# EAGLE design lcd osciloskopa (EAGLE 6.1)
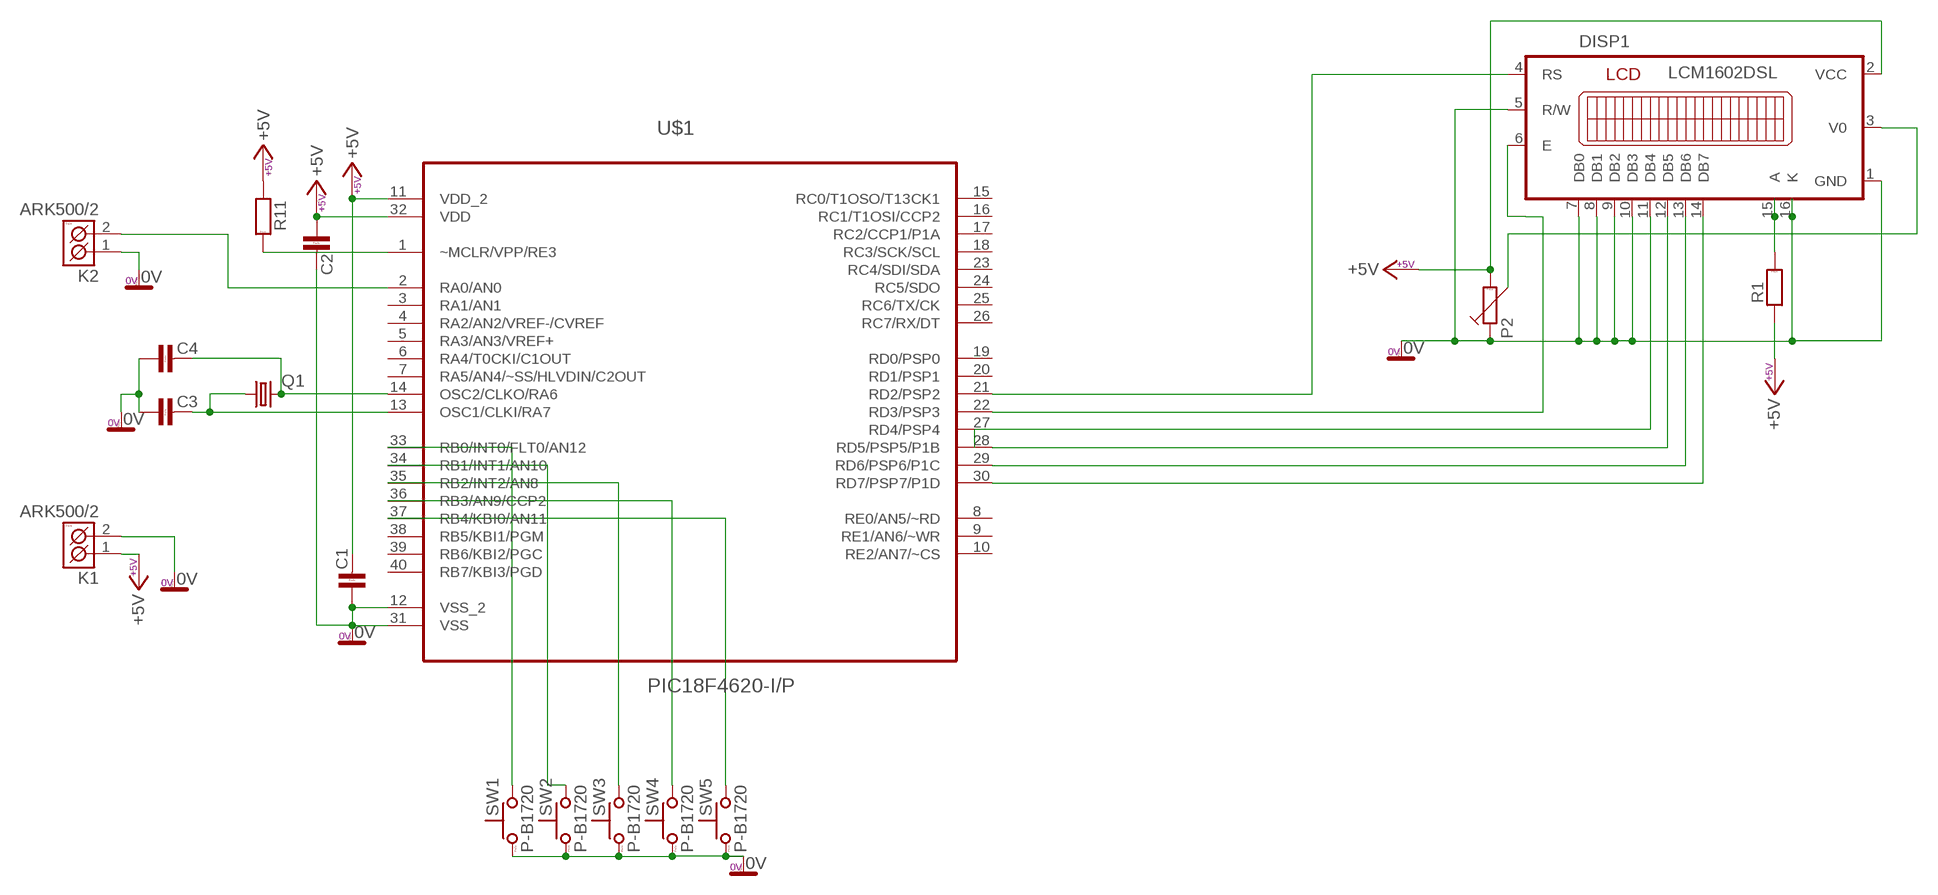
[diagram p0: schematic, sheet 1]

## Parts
C1  C-KERAMIK_7,5  [C-7,5]
C2  C-KERAMIK_7,5  [C-7,5]
C3  C-KERAMIK_7,5  [C-7,5]
C4  C-KERAMIK_7,5  [C-7,5]
DISP1  LCM1602DSL  [LCM1602DSL]
K1  ARK500/2  [ARK500/2]
K2  ARK500/2  [ARK500/2]
P2  TRIMRPT10V  [PT10V]
Q1  CRYSTALHC49U70  [HC49U70]
R1  R_7,5  [R-7,5]
R11  R_7,5  [R-7,5]
SW1  P-B1720  [P-B1720]
SW2  P-B1720  [P-B1720]
SW3  P-B1720  [P-B1720]
SW4  P-B1720  [P-B1720]
SW5  P-B1720  [P-B1720]
U$1  PIC18F4620-I/P  [DIP254P1524X635-40]

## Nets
+5V: C1.2 C2.1 DISP1.2(VCC) K1.1(K1) P2.2 R1.1 R11.1 U$1.11(VDD_2) U$1.32(VDD)
N$1: DISP1.4(RS) U$1.21(RD2/PSP2)
N$2: DISP1.6(E) U$1.22(RD3/PSP3)
N$3: DISP1.14(DB7) U$1.30(RD7/PSP7/P1D)
N$4: DISP1.13(DB6) U$1.29(RD6/PSP6/P1C)
N$5: DISP1.12(DB5) U$1.28(RD5/PSP5/P1B)
N$6: DISP1.11(DB4)
N$8: DISP1.3(V0) P2.3
N$9: SW5.2 U$1.37(RB4/KBI0/AN11)
N$10: SW4.2 U$1.36(RB3/AN9/CCP2)
N$11: SW3.2 U$1.35(RB2/INT2/AN8)
N$12: SW2.2 U$1.34(RB1/INT1/AN10)
N$13: SW1.2 U$1.33(RB0/INT0/FLT0/AN12)
N$17: K2.2(K2) U$1.2(RA0/AN0)
N$20: R11.2 U$1.1(~MCLR/VPP/RE3)
N$51: C3.2 Q1.1 U$1.13(OSC1/CLKI/RA7)
N$55: C4.2 Q1.2 U$1.14(OSC2/CLKO/RA6)
N$56: C1.1 C2.2 C3.1 C4.1 DISP1.1(GND) DISP1.5(R/W) DISP1.7(DB0) DISP1.8(DB1) DISP1.9(DB2) DISP1.10(DB3) DISP1.16(K) K1.2(K2) K2.1(K1) P2.1 SW1.1 SW2.1 SW3.1 SW4.1 SW5.1 U$1.12(VSS_2) U$1.31(VSS) ; supply symbol labelled 0V
N$57: DISP1.15(A) R1.2
Unconnected: SW1.3 SW1.4 SW2.3 SW2.4 SW3.3 SW3.4 SW4.3 SW4.4 SW5.3 SW5.4 U$1.3(RA1/AN1) U$1.4(RA2/AN2/VREF-/CVREF) U$1.5(RA3/AN3/VREF+) U$1.6(RA4/T0CKI/C1OUT) U$1.7(RA5/AN4/~SS/HLVDIN/C2OUT) U$1.8(RE0/AN5/~RD) U$1.9(RE1/AN6/~WR) U$1.10(RE2/AN7/~CS) U$1.15(RC0/T1OSO/T13CK1) U$1.16(RC1/T1OSI/CCP2) U$1.17(RC2/CCP1/P1A) U$1.18(RC3/SCK/SCL) U$1.19(RD0/PSP0) U$1.20(RD1/PSP1) U$1.23(RC4/SDI/SDA) U$1.24(RC5/SDO) U$1.25(RC6/TX/CK) U$1.26(RC7/RX/DT) U$1.27(RD4/PSP4) U$1.38(RB5/KBI1/PGM) U$1.39(RB6/KBI2/PGC) U$1.40(RB7/KBI3/PGD)

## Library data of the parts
C1-C4 = #PaJa_30:C-KERAMIK: Kondenzator - keramicky
DISP1 = #PaJa_displeje:LCM1602DSL: LCD - 2x16 + LED (TME - LCM1602DSL)
K1 K2 = #PaJa_konektory:ARK500/2: Svorkovnice - roztec 5mm - dvojita
P2 = #PaJa_30:TRIMR: Trimr
Q1 = crystal:CRYSTAL: CRYSTAL; OC_FARNELL: unknown; OC_NEWARK: unknown
R1 R11 = #PaJa_30:R: Rezistor
SW1-SW5 = #PaJa_prepinace:P-B1720: &micro;-tlacitko
U$1 = PIC18F4620:PIC18F4620-I/P: Flash Microcontrollers; MPN: PIC18F4620-I/P; OC_FARNELL: 1212704; OC_NEWARK: 89H0709; PACKAGE: DIP-40; SUPPLIER: Microchip

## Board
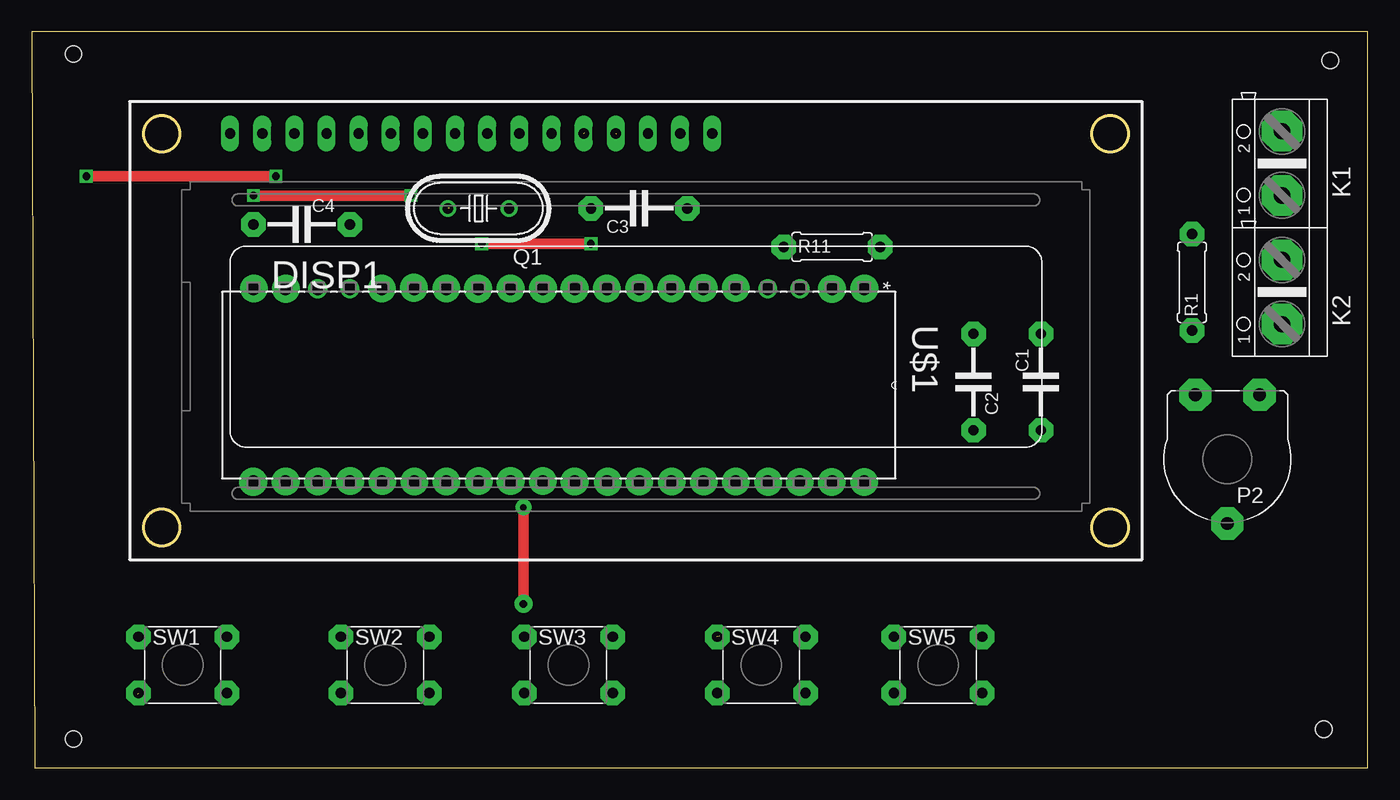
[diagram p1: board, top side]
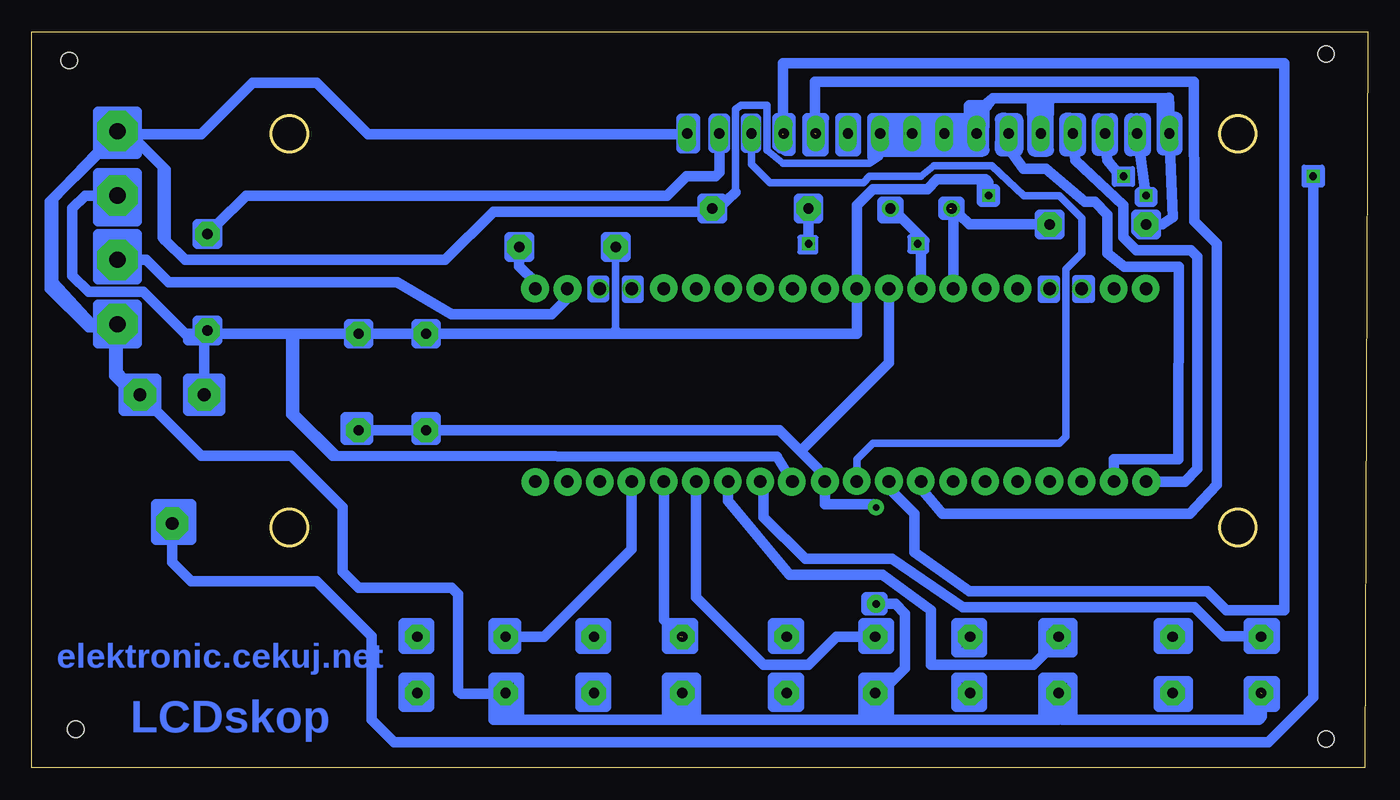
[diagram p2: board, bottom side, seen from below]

Size 105.59 x 58.16 mm. Coordinates in mm from the lower left corner, seen from the top.
Outline: 0.25,0 105.59,0 105.59,58.16 0,58.16 0.25,0
Copper layers (1*16): Top 0.035mm / dielectric 1.5mm / Bottom 0.035mm
Design rules: minimum track width 10mil, minimum drill 24mil, track to track 8mil, track to pad 8mil, pad to pad 8mil, via to via 8mil, smd to smd 8mil, copper to edge 40mil, drill to drill 8mil, minimum pad ring 10mil, minimum via ring 8mil, stop-mask expansion 4mil, vias tented up to drill 0mil, thermal gap 10mil
Holes 1.3 mm at 3.3,56.39 3.3,2.29 102.11,3.05 102.62,55.88

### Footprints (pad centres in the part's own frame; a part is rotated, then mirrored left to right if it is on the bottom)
C-7,5 = drill 0.813 pad 1.93 octagon: 1 -3.81,0; 2 3.81,0
LCM1602DSL = drill 0.813 pad 1.422 long: 1 -32.068,16.828; 2 -29.527,16.828; 3 -26.988,16.828; 4 -24.448,16.828; 5 -21.907,16.828; 6 -19.367,16.828; 7 -16.828,16.828; 8 -14.287,16.828; 9 -11.748,16.828; 10 -9.207,16.828; 11 -6.668,16.828; 12 -4.128,16.828; 13 -1.587,16.828; 14 0.953,16.828; 15 3.493,16.828; 16 6.032,16.828 | hole 2.8: -37.465,-14.287; 37.465,-14.287; 37.465,16.828; -37.465,16.828
ARK500/2 = drill 1.27 pad 3.2 octagon: 1 -2.54,0; 2 2.54,0
PT10V = drill 1.016 pad 2.54 octagon: 1 -2.54,-5.08; 2 2.54,-5.08; 3 0,5.08
HC49U70 = drill 0.813: 1 -2.413,0; 2 2.413,0
R-7,5 = drill 0.813 pad 1.93 octagon: 1 -3.81,0; 2 3.81,0
P-B1720 = drill 0.813 pad 1.93 octagon: 1 -3.493,-2.223; 2 -3.493,2.223; 3 3.493,-2.223; 4 3.493,2.223
DIP254P1524X635-40 = drill 0.991 square: 1 -15.24,48.26 | drill 0.991: 2 -15.24,45.72; 3 -15.24,43.18; 4 -15.24,40.64; 5 -15.24,38.1; 6 -15.24,35.56; 7 -15.24,33.02; 8 -15.24,30.48; 9 -15.24,27.94; 10 -15.24,25.4; 11 -15.24,22.86; 12 -15.24,20.32; 13 -15.24,17.78; 14 -15.24,15.24; 15 -15.24,12.7; 16 -15.24,10.16; 17 -15.24,7.62; 18 -15.24,5.08; 19 -15.24,2.54; 20 -15.24,0; 21 0,0; 22 0,2.54; 23 0,5.08; 24 0,7.62; 25 0,10.16; 26 0,12.7; 27 0,15.24; 28 0,17.78; 29 0,20.32; 30 0,22.86; 31 0,25.4; 32 0,27.94; 33 0,30.48; 34 0,33.02; 35 0,35.56; 36 0,38.1; 37 0,40.64; 38 0,43.18; 39 0,45.72; 40 0,48.26

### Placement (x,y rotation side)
C1  79.76,30.48 90 top
C2  74.42,30.48 270 top
C3  48.01,44.2 180 top
C4  21.34,42.93 0 top
DISP1  47.75,33.27 0 top
K1  98.81,47.75 90 top
K2  98.81,37.59 90 top
P2  94.49,24.38 180 top
Q1  35.31,44.2 180 top
R1  91.69,38.35 90 top
R11  63.25,41.15 0 top
SW1  11.94,8.13 0 top
SW2  27.94,8.13 0 top
SW3  42.42,8.13 0 top
SW4  57.66,8.13 0 top
SW5  71.63,8.13 0 top
U$1  17.53,22.61 270 top

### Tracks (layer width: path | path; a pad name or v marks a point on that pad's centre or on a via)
+5V  (via drill 0.5 pad 2.18, 0.6)
  Top 0.813: v17.53,45.21 v29.97,45.21
  Bottom 0.254: 92.46,34.04 R1.1 | 98.81,44.2 98.81,44.96 K1.1
  Bottom 0.61: R11.1 59.44,34.54 | C2.1 74.68,34.29
  Bottom 0.813: C1.2 74.68,34.29 74.42,34.54 C2.1 | 84.84,34.29 91.44,34.29 R1.1 | 92.46,34.04 92.96,34.04 | 93.22,34.04 96.77,37.59 101.09,37.59 102.36,38.86 102.36,44.2 101.35,45.21 99.06,45.21 98.81,44.96 | 91.95,30.73 91.95,34.29 R1.1 | 45.72,22.61 v45.52,22.61 U$1.32 46.71,24.59 81.53,24.64 | 59.44,34.54 59.69,34.29 C2.1 | 80.01,34.54 C1.2 | C1.2 84.84,34.29 | 84.84,34.29 85.09,34.04 85.09,27.94 81.79,24.64 81.53,24.64 | DISP1.2 v17.53,45.21 17.53,45.47 17.78,45.47 17.78,44.96 17.27,44.96 | U$1.11 40.39,44.45 39.12,45.72 34.8,45.72 34.04,46.48 30.23,46.48 29.97,46.23 29.97,45.72 | U$1.11 v40.41,37.85 40.64,37.85 | 81.53,24.64 84.84,27.94 84.84,34.29 | C1.2 C2.1 | C2.1 40.39,34.29 U$1.11 | P2.2 91.95,30.73 | 91.95,30.73 93.22,30.73 93.22,28.19 90.68,28.19 90.68,30.73 91.95,30.73 | R1.1 91.69,35.31 | 91.69,35.31 92.46,35.31 92.46,33.78 | 92.46,33.78 90.93,33.78 90.93,35.31 91.69,35.31 | 92.46,33.78 92.96,33.78 | 92.96,33.78 93.22,33.78 93.22,34.04 | 93.22,34.04 92.96,34.04 | 92.96,34.04 92.96,34.29 93.22,34.29 | 92.96,34.04 92.96,33.78 | C2.1 74.42,35.05 | 74.42,35.05 75.18,35.05 75.18,33.53 73.66,33.53 73.66,35.05 74.42,35.05 | C1.2 79.76,35.05 | 79.76,35.05 78.99,35.05 78.99,33.53 80.52,33.53 80.52,35.05 79.76,35.05 | R11.1 59.44,41.91 | 59.44,41.91 60.2,41.91 60.2,40.39 58.67,40.39 58.67,41.91 59.44,41.91 | v29.97,45.21 29.97,45.72 | 29.97,45.72 30.48,45.72 | 30.48,45.72 30.48,44.7 29.46,44.7 29.46,45.72 29.97,45.72 | 30.48,46.23 30.48,45.72 | 17.27,44.96 17.27,45.47 | 17.27,44.96 17.27,44.7 18.03,44.7 18.03,45.47 17.02,45.47 17.02,44.7
N$1  (via drill 0.5 pad 2.18)
  Bottom 0.813: 23.37,50.04 23.11,48.01 19.3,44.45 19.3,41.91 18.29,40.89 13.97,40.89 13.46,40.39 13.46,23.62 14.48,22.61 v17.5,22.61 U$1.21 | 23.37,50.04 23.11,50.04 | DISP1.4 23.37,50.04
N$2  (via drill 0.5 pad 2.18)
  Bottom 0.813: 28.19,49.28 28.26,50.1 DISP1.6 28.45,50.04 28.45,49.02 27.2,47.32 25.43,47.32 22.35,44.7 21.59,44.7 20.57,43.69 20.57,40.64 19.25,39.6 14.93,39.6 14.99,24.38 20.07,24.38 v20.07,22.63 U$1.22
N$3  (via drill 0.5 pad 2.18)
  Bottom 0.61: DISP1.14 48.7,47.69 47.24,46.23 39.88,46.23 39.37,46.74 35.31,46.74 34.29,47.57 29.72,47.57 27.18,45.21 24.38,45.21 22.61,43.43 22.61,40.64 23.88,39.37 23.88,26.16 24.38,25.65 39.12,25.65 40.39,24.38 v40.39,22.66 U$1.30
N$4  (1 unrouted)
  Bottom 0.813: U$1.29 37.85,22.1 35.81,20.07 35.81,17.02 31.5,13.97 12.7,13.97 11.18,12.45 6.6,12.45 6.6,55.68 46.23,55.68 46.23,50.04 46.48,49.78
N$5  (1 unrouted)
  Bottom 0.813: U$1.28 35.31,22.1 33.63,20.09 14.07,20.09 11.94,22.35 11.94,41.4 13.72,43.18 13.77,53.34 13.77,54.2 43.69,54.2 43.69,50.11 | 43.69,50.11 43.69,49.78 | 43.69,50.11 44.09,50.11 44.09,51.26
N$7
  Bottom 0.813: 44.2,44.45 44.2,44.96 | 44.2,44.96 44.96,44.96 44.96,43.43 43.43,43.43 43.43,44.96 44.2,44.96
N$8  (via drill 0.6)
  Top 0.813: v4.32,46.74 v19.3,46.74
  Bottom 0.813: v4.32,46.74 4.32,5.59 7.87,2.03 76.96,2.03 78.74,3.81 78.74,10.41 83.06,14.73 92.96,14.73 94.49,16.26 P2.3 94.49,20.57 | DISP1.3 20.83,50.04 20.57,48.01 19.56,46.74 v19.3,46.74 19.3,46.99 | 94.49,20.83 95.76,20.83 95.76,20.07 | 95.76,20.07 95.76,18.03 93.73,18.03 | 93.47,18.03 92.96,18.03 92.96,20.83 94.49,20.83 | 94.49,20.83 94.49,20.57 | 94.49,20.57 93.22,20.57 93.22,20.07 93.73,20.07 | 95.76,20.07 93.73,20.07 | 93.73,20.07 93.73,18.03 | 93.73,18.03 93.47,18.03 | 93.47,18.03 93.47,18.29 94.74,18.29 94.74,18.54 | 19.3,46.99 19.81,46.99 19.81,46.48 18.8,46.48 18.8,46.99 19.3,46.99
N$9
  Bottom 0.813: SW5.2 65.09,10.35 58.17,17.27 U$1.37
N$10  (1 unrouted)
  Bottom 0.813: U$1.36 55.63,11.68 54.36,10.41
N$11
  Bottom 0.813: U$1.35 53.09,14.48 53.09,14.22 53.09,13.46 47.75,8.13 44.2,8.13 41.97,10.35 SW3.2
N$12
  Bottom 0.813: U$1.34 50.55,21.08 45.72,15.24 38.35,15.24 34.54,12.45 34.54,8.13 26.42,8.13 24.38,10.16 24.45,10.22 SW2.2
N$13
  Bottom 0.813: U$1.33 47.75,22.86 47.75,19.81 44.45,16.51 37.59,16.51 32,12.7 13.72,12.7 11.43,10.41 8.64,10.41 | 8.64,10.41 8.64,11.43 | 8.64,11.43 9.4,11.43 9.4,9.4 7.62,9.4 | 7.62,9.4 7.62,11.43 | 7.62,11.43 8.13,11.43 8.64,11.43 | SW1.2 8.57,10.35 8.64,10.41 | 7.62,9.4 7.37,9.4 7.37,11.43 7.62,11.43
N$14
  Bottom 0.813: 25.15,43.18 25.15,43.69 | 25.15,43.69 25.91,43.69 25.91,42.16 24.38,42.16 24.38,43.69 25.15,43.69
N$15  (via drill 0.6 pad 1.42)
  other vias: 38.86,12.95
N$16
  Bottom 0.813: 51.21,49.02 50.8,49.02 | 50.8,49.02 50.8,49 | 50.8,49.02 50.8,51.28 51.66,51.28 51.66,51.21 51.69,51.21 51.69,49 51.11,49
N$17  (via drill 0.5 pad 2.18)
  Bottom 0.813: U$1.2 v63.25,37.82 63.25,37.08 64.52,35.81 72.39,35.81 76.71,38.35 94.74,38.35 96.52,40.13 K2.2 99.06,40.39
N$18  (via drill 0.5 pad 1.27)
  other vias: 38.86,20.57
N$20
  Bottom 0.813: U$1.1 65.79,38.35 67.06,39.62 67.06,40.64 67.06,40.89 | 67.06,40.89 67.31,41.15 R11.2 | 67.06,40.89 R11.2 | R11.2 67.06,41.91 | 67.06,41.91 66.29,41.91 66.29,40.39 67.82,40.39 67.82,41.91 67.06,41.91 | 67.06,40.89 R11.2
N$23
  Bottom 0.813: 8.89,10.92 8.89,11.18
N$24
  Bottom 0.813: 8.13,10.67 8.38,10.67 8.38,10.16 8.38,9.91
N$25
  Bottom 0.813: 8.13,10.41 8.64,10.41 8.64,10.16
N$26
  Bottom 0.813: 8.64,5.84 8.64,6.86 9.4,6.86 9.4,4.32 8.89,4.32 8.89,4.83
N$27
  Bottom 0.813: 8.64,4.83 7.37,4.83 7.37,6.86 8.38,6.86
N$28
  Bottom 0.813: 15.49,10.41 15.49,11.43 14.22,11.43 14.22,9.4 16.51,9.4 16.51,11.43 14.99,11.43 14.99,11.18
N$29
  Bottom 0.813: 14.99,10.16 15.49,10.16 15.49,9.91
N$30
  Bottom 0.813: 61.21,10.41 61.21,11.43 | 61.21,11.43 60.2,11.43 60.2,9.4 61.47,9.4 61.98,9.4 | 61.98,9.4 61.98,11.43 | 61.98,11.43 61.21,11.43 | 61.98,11.43 62.23,11.43 62.23,9.4 61.98,9.4
N$31
  Bottom 0.813: 14.48,6.1 14.73,6.1 14.73,5.33 15.49,5.33 | 15.49,5.33 16,5.33 16,6.1 14.99,6.1 14.99,6.35 15.49,6.35 15.49,6.1 15.49,5.33 | 15.49,4.83 14.22,4.83 14.22,6.86 16.51,6.86 16.51,4.83 15.49,4.83 | 15.49,4.83 15.49,5.33
N$32
  Bottom 0.813: 24.38,10.41 23.37,10.41 | 23.37,10.41 23.37,10.92 23.37,11.18 23.37,11.43 25.65,11.43 25.65,9.14 23.37,9.14 23.37,10.41
N$33
  Bottom 0.813: 24.64,6.1 24.64,7.11 | 25.15,7.11 25.65,7.11 25.65,5.08 | 25.65,5.08 24.64,5.08 | 24.64,5.08 23.37,5.08 23.37,7.11 24.64,7.11 | 24.64,7.11 25.15,7.11 | 25.15,7.11 25.15,6.1 24.89,6.1 24.89,5.33 | 25.65,5.08 25.65,4.32 23.37,4.32 23.37,4.83 24.64,4.83 24.64,5.08
N$34
  Bottom 0.813: 31.5,10.41 31.5,11.43 30.48,11.43 30.48,9.14 32.51,9.14 32.51,11.43 31.24,11.43 31.24,11.18
N$35
  Bottom 0.813: 31.24,10.41 31.5,10.41 31.5,9.91
N$36
  Bottom 0.813: 31.5,5.84 31.5,7.11 | 31.5,7.11 30.48,7.11 30.48,5.08 | 30.48,5.08 32.51,5.08 | 32.51,5.08 32.51,5.33 32.51,7.11 31.5,7.11 | 30.48,5.08 30.48,4.83 32.51,4.83 32.51,5.08
N$37
  Bottom 0.813: 39.12,10.41 38.86,10.41 38.86,11.43 37.85,11.43 37.85,9.4 39.88,9.4 39.88,11.43 39.12,11.43 39.12,11.18 39.12,10.92
N$38
  Bottom 0.813: 38.86,12.7 39.12,12.7 39.12,12.95
N$39
  Bottom 0.813: 45.97,5.84 45.97,7.11 | 45.97,7.11 44.96,7.11 44.96,4.83 46.23,4.83 46.74,4.83 | 46.74,4.83 46.74,7.11 | 46.74,7.11 45.97,7.11 | 46.74,7.11 46.99,7.11 46.99,4.83 46.74,4.83
N$40
  Bottom 0.813: 45.97,10.41 45.97,11.43 | 45.97,11.43 44.96,11.43 44.96,9.4 46.74,9.4 46.74,11.43 | 46.74,11.43 45.97,11.43 | 46.74,11.43 46.99,11.43 46.99,9.4
N$41
  Bottom 0.813: 54.1,6.1 54.1,7.11 | 54.1,7.11 53.59,7.11 53.34,7.11 | 53.34,7.11 53.34,4.32 | 53.34,4.32 55.12,4.32 55.12,7.11 | 55.12,7.11 54.1,7.11 | 55.12,7.11 55.37,7.11 55.37,4.32 | 53.34,4.32 53.09,4.32 53.09,7.11 53.34,7.11
N$42
  Bottom 0.813: 54.1,10.41 54.1,11.43 | 54.1,11.43 54.86,11.43 55.12,11.43 | 55.12,11.43 55.12,9.4 53.34,9.4 53.34,11.43 54.1,11.43 | 55.12,11.43 55.37,11.43 55.37,9.4
N$43
  Bottom 0.813: 61.21,6.1 61.21,7.11 62.23,7.11 62.23,4.83 60.2,4.83 60.2,7.11 61.47,7.11 61.47,5.59
N$44
  Bottom 0.813: 60.96,5.33 60.71,5.33 60.71,5.84 61.21,5.84 61.21,5.08
N$45
  Bottom 0.813: 68.07,10.41 68.07,11.43 | 68.07,11.43 67.31,11.43 67.31,9.4 69.09,9.4 69.09,11.43 68.07,11.43
N$46
  Bottom 0.813: 74.93,10.16 74.93,10.41 | 74.93,10.41 74.93,11.43 | 74.93,11.43 74.17,11.43 74.17,9.4 75.18,9.4 | 75.18,9.4 75.95,9.4 | 75.95,9.4 75.95,11.43 75.18,11.43 | 74.93,11.43 76.2,11.43 76.2,9.4 75.95,9.4 | 75.18,9.4 75.18,10.16 | 74.93,10.41 75.44,10.41 75.44,10.92 74.93,10.92 74.93,9.91
N$47
  Bottom 0.813: 75.18,5.84 75.18,7.11 | 75.18,7.11 74.93,7.11 74.17,7.11 74.17,4.83 76.2,4.83 76.2,7.11 75.18,7.11
N$48
  Bottom 0.813: 91.69,29.21 91.19,29.21 91.19,29.97 92.2,29.97 92.2,28.96 91.95,28.96
N$49
  Bottom 0.813: 90.93,28.7 92.71,28.7 92.71,30.23 92.96,30.23 92.96,29.72
N$50
  Bottom 0.813: 98.3,44.96 98.3,45.72
N$51  (via drill 0.6)
  Top 0.813: v44.2,41.4 v35.56,41.4
  Bottom 0.406: 44.25,41.45 44.2,41.45 44.2,41.91 | 44.2,41.91 44.83,41.91 | 44.83,41.91 44.88,41.91 44.88,40.77 43.61,40.77 43.61,41.86 44.83,41.86 44.83,41.91 | 44.2,41.91 43.61,41.91 43.61,41.88 44.02,41.88 44.02,41.4
  Bottom 0.813: 37.59,43.94 37.85,43.94 37.85,44.7 | 37.85,44.7 37.08,44.7 37.08,43.69 | U$1.13 35.31,41.91 | C3.2 44.2,41.91 v44.2,41.4 | v35.56,41.4 35.05,41.66 35.31,41.91 | 35.31,41.91 37.08,43.69 | 37.08,43.69 37.59,44.2 Q1.1 | 37.08,43.69 37.08,43.43 38.35,43.43 38.35,44.7 37.85,44.7
N$52
  Bottom 0.813: 98.81,39.88 98.81,41.66 100.33,41.66 | 100.33,41.66 100.33,38.61 97.28,38.61 97.28,41.66 | 97.28,41.66 98.55,41.66 | 97.28,41.66 97.28,42.16 100.33,42.16 100.33,41.66
N$53
  Bottom 0.813: 99.31,40.13 99.06,40.13 99.06,39.37 98.55,39.37 | 98.55,39.37 98.3,39.37 98.3,39.62 98.55,39.62 98.55,39.37
N$54
  Bottom 0.813: 98.81,45.47 98.81,46.74 100.08,46.74 100.08,43.69 | 100.08,43.69 97.54,43.69 | 97.54,43.69 97.54,46.74 99.06,46.74 99.06,46.48 | 97.54,43.69 97.54,43.43 | 97.54,43.18 100.08,43.18 100.08,43.69 | 98.04,43.43 97.54,43.43 | 97.54,43.43 97.54,43.18 | 97.54,43.18 97.28,43.18 97.28,46.74 | 97.28,46.74 100.33,46.74 | 100.33,46.74 100.33,43.18 | 97.28,46.74 97.28,46.99 100.33,46.99 100.33,46.74
N$55  (via drill 0.5 pad 2.18)  (1 unrouted)
  Bottom 0.813: 33.02,44.2 33.02,44.7 32.26,44.7 32.26,43.69 | C4.2 31.5,42.93 32.26,43.69 | 32.26,43.69 32.77,44.2 v32.77,37.87 U$1.14 | 32.26,43.69 33.27,43.69 33.27,44.7 33.53,44.7 33.53,43.69
N$56  (via drill 0.5 pad 1.27)  (1 unrouted)
  Top 0.813: v38.86,20.57 v38.86,12.95
  Bottom 0.254: 54.36,6.1 SW4.1 | 68.33,6.1 SW5.1 | 53.85,50.04 DISP1.16 | 98.81,49.28 98.81,49.78 98.81,50.04 K1.2 | 100.08,34.04 98.81,34.04 98.81,34.29 K2.1
  Bottom 0.61: 49.99,45.47 49.96,52.05 49.53,52.32 47.5,52.32 47.5,48.77 46.23,47.75 39.37,47.75 38.61,48.26 38.61,50.04 DISP1.10
  Bottom 0.813: 98.55,50.8 99.57,50.8 99.57,50.29 98.3,50.29 98.3,49.78 98.04,49.78 98.04,48.77 | 98.81,50.55 98.81,51.82 | 98.81,51.82 100.33,51.82 100.33,48.77 98.55,48.77 | 98.04,48.77 97.54,48.77 97.54,51.56 | 97.54,51.56 97.54,51.82 98.81,51.82 | 97.54,51.56 97.28,51.56 | 97.28,51.56 97.28,51.82 | 97.28,51.56 97.28,48.51 98.55,48.51 | 100.08,34.8 100.08,36.32 | 100.08,36.58 97.28,36.58 97.28,33.53 100.08,33.53 100.08,34.8 | 96.52,29.97 97.54,29.97 97.54,28.45 96.77,28.45 96.77,28.7 96.01,28.7 96.01,29.72 96.77,29.72 96.77,29.21 | 68.07,3.81 68.07,5.91 SW5.1 68.2,5.84 68.33,5.84 | 68.07,3.81 54.36,3.81 | 54.36,3.81 54.17,3.81 | 54.17,3.81 SW4.1 54.36,5.91 54.36,3.81 | 54.17,3.81 38.93,3.81 SW3.1 38.86,5.91 | 38.86,5.91 38.86,5.84 | 38.86,5.84 38.86,3.81 24.45,3.81 SW2.1 24.45,4.13 24.13,3.81 8.64,3.81 8.38,4.06 8.38,5.84 | v38.86,20.57 39.12,20.83 42.9,20.83 42.9,22.89 42.93,22.89 U$1.31 42.75,22.66 43.51,23.67 43.69,23.88 44.83,25.02 | 38.86,5.84 38.61,6.1 38.35,6.1 36.58,7.87 36.58,12.19 37.34,12.95 v38.86,12.95 38.86,13.46 39.62,13.46 39.62,12.45 38.35,12.45 38.35,13.46 38.61,13.46 | 25.6,52.91 25.91,50.16 | 25.91,50.16 DISP1.5 26.1,52.13 25.6,52.91 | 38.61,50.04 38.35,50.04 38.42,50.1 DISP1.10 DISP1.9 DISP1.8 DISP1.7 30.91,50.1 30.91,50.67 | 98.3,50.04 98.81,49.78 | 98.81,34.04 98.81,31.24 98.3,30.73 | 98.3,30.73 P2.1 97.03,29.97 | C2.2 79.5,26.67 79.76,26.42 80.01,26.67 C1.1 | C1.1 C2.2 | C2.2 46.48,26.67 44.83,25.02 | 25.6,52.91 15.72,52.93 15.68,52.26 DISP1.1 15.43,43.5 16.26,42.93 C4.1 17.53,43.69 | K2.1 100.84,35.05 103.89,38.35 103.89,44.96 K1.2 | 98.3,50.04 98.81,50.04 99.31,50.04 99.31,49.53 100.33,48.51
  Bottom 0.813: 98.3,50.04 97.79,50.04 | 95.25,47.5 95.25,41.91 95,41.66 | C3.1 52.07,43.94 69.09,43.94 72.9,40.13 93.47,40.13 95,41.66 | C3.1 51.31,44.2 49.99,45.47 | 95,41.66 95,47.24 95.25,47.5 | 95.25,47.5 97.79,50.04 | 100.33,48.51 104.14,44.7 104.14,37.85 101.09,34.8 100.33,34.8 | 100.08,34.8 99.06,34.8 | 99.06,34.8 99.06,34.54 | 99.06,34.54 99.06,30.99 97.28,29.21 96.77,29.21 | 96.77,29.21 95.76,28.19 | 95.76,28.19 92.2,24.64 85.09,24.64 81.03,20.57 81.03,15.49 79.76,14.22 72.39,14.22 71.88,13.72 71.88,6.1 71.63,5.84 68.33,5.84 | U$1.12 37.85,32 44.83,25.02 | 53.85,50.04 78.99,50.04 83.06,54.1 88.14,54.1 92.2,50.04 97.79,50.04 | 38.86,5.91 38.86,7.11 | 38.86,7.11 38.61,7.11 | 38.61,7.11 38.1,7.11 | 38.1,7.11 37.59,7.11 | 38.1,7.11 38.1,4.32 37.85,4.32 37.85,6.35 38.61,6.35 38.61,7.11 | 38.86,7.11 39.88,7.11 39.88,4.32 39.12,4.32 39.12,4.83 39.37,4.83 39.37,6.35 | 68.33,5.84 68.33,7.11 | 68.33,7.11 67.06,7.11 67.06,5.08 | 67.06,4.83 67.06,4.32 69.09,4.32 | 69.09,4.32 69.09,7.11 68.33,7.11 | 68.33,5.84 68.33,4.83 67.06,4.83 | 67.06,4.83 67.06,5.08 | 67.06,5.08 67.31,5.08 | 68.07,3.81 69.09,3.81 69.09,4.32 | C1.1 79.76,27.69 80.77,27.69 80.77,25.91 78.99,25.91 78.99,27.69 79.5,27.69 | C2.2 74.42,27.69 75.18,27.69 75.18,25.91 73.66,25.91 73.66,27.69 74.17,27.69 | 97.03,29.97 97.03,30.73 | 97.03,30.73 95.76,30.73 95.76,28.19 | 95.76,28.19 98.3,28.19 98.3,30.73 | 98.3,30.73 97.03,30.73 | 96.77,29.21 96.27,29.21 96.27,29.97 97.03,29.97 | 100.08,34.8 100.33,34.8 | 100.33,34.8 100.33,36.58 100.08,36.58 | 100.08,36.58 100.08,36.32 | 100.08,36.32 100.33,36.32 100.33,33.53 98.3,33.53 98.3,35.56 99.06,35.56 99.06,34.8
  Bottom 0.813: 99.06,34.54 98.81,34.54 98.81,34.29 | 100.33,48.51 98.55,48.51 | 98.55,48.51 98.55,49.53 | 98.04,48.77 98.55,48.77 | 98.55,48.77 98.55,50.55 | C3.1 51.82,44.96 | 51.82,44.96 52.58,44.96 52.58,43.43 51.05,43.43 51.05,44.96 51.82,44.96 | 17.53,43.69 18.29,43.69 18.29,42.42 18.03,42.16 16.76,42.16 16.76,43.69 17.53,43.69 | 25.91,50.16 25.73,50.16 25.73,52.3 25.86,52.3 25.45,52.91 29.62,52.91 | 29.62,52.91 30.3,52.32 | 30.3,52.32 30.3,50.67 30.91,50.67 | 30.91,50.67 31.04,50.67 31.04,50.09 | 30.1,52.25 30.1,52.3 29.62,52.91 | 30.3,52.32 31.5,52.32 31.52,52.3 31.52,50.34 31.62,50.24 31.62,51.28 30.94,51.97 30.94,50.98 31.04,50.88 31.04,51.44 31.01,51.44 30.81,51.23 30.81,51.28 30.79,51.31 | 30.46,51.21 30.56,51.21 30.56,51.11 30.58,51.11 30.58,51.41 | 30.46,51.74 30.4,51.74 30.4,51.69 30.38,51.69 30.38,51.41 30.58,51.41 | 30.58,51.41 30.61,51.41 30.73,51.41 30.73,51.03 30.76,51.03 30.76,50.62 | 30.61,51.31 30.79,51.31 | 30.79,51.31 30.94,51.31 30.94,50.44 30.96,50.44 30.96,50.11 30.91,50.11 30.91,50.14 30.81,50.14 30.81,50.49 | 30.79,51.31 30.79,51.33 39.14,51.33 39.14,49.78 | 39.14,48.26 39.14,49.78 | 39.14,49.78 37.92,51 37.92,50.65 37.8,50.52 32.49,50.52 32.26,50.75 32.26,50.6 31.04,49.38 37.64,49.38 37.85,49.58
  Bottom 1.016: 30.96,51.13 30.94,51.16 30.4,51.16 | 38.96,51.16 38.99,51.13 38.99,48.82 38.96,48.79 30.4,48.79 30.4,51.16 | 30.58,51.44 30.61,51.41 30.61,51.31 30.61,51.28 30.46,51.13 30.46,51.21 30.4,51.16
N$57
  Bottom 0.813: 91.69,42.42 91.69,42.93 | 91.69,42.93 92.46,42.93 92.46,41.4 90.93,41.4 90.93,42.93 | DISP1.15 51.25,47.05 51.56,46.74 53.85,46.74 55.37,45.21 88.65,45.21 90.93,42.93 | 90.93,42.93 R1.2 | 90.93,42.93 91.19,42.93 91.44,42.93 91.69,42.93
N$58
  Bottom 0.813: 53.77,50.09 53.77,51.26 53.19,51.26 53.19,48.95 54.23,48.95 54.23,51.21 53.85,51.21 | 53.8,51.21 53.85,51.21 | 53.85,51.21 53.85,51.26 | 53.85,51.26 54.23,51.26 | 53.85,51.26 53.75,51.26 53.75,51.16 | 53.75,51.13 53.75,51.16 | 53.75,51.16 53.7,51.16 53.7,50.16
N$59
  Bottom 0.813: 48.72,50.11 48.72,51.26 49.12,51.26 49.12,49 48.34,49
N$60
  Bottom 0.813: 48.34,49.05 48.34,51.26 48.77,51.26 48.77,51.23
N$61
  Bottom 0.813: 46.15,50.09 46.18,50.09 46.18,51.26 46.58,51.26 46.58,49.12 46.41,49.12 46.41,48.95 45.72,48.95 45.72,51.23 46.33,51.23
N$62
  Bottom 0.813: 43.51,50.01 43.59,50.01 43.59,51.23 44.12,51.23 44.12,51.26 44.15,51.26 44.15,49 43.16,49 43.16,51.16 43.48,51.16 43.48,51.18
N$63
  Bottom 0.813: 41.07,50.19 41.05,50.19 41.05,51.21
N$64  (via drill 0.5 pad 2.18)
  other vias: 65.79,22.58
N$65  (via drill 0.5 pad 2.18)
  other vias: 63.22,22.58
N$66  (via drill 0.5 pad 2.18)
  other vias: 60.71,22.58
N$67  (via drill 0.5 pad 2.18)
  other vias: 58.19,22.61
N$68  (via drill 0.5 pad 2.18)
  other vias: 55.63,22.63
N$69  (via drill 0.5 pad 2.18)
  other vias: 53.11,22.63
N$70  (via drill 0.5 pad 2.18)
  other vias: 50.57,22.63
N$71  (via drill 0.5 pad 2.18)
  other vias: 48.01,22.63
N$72  (via drill 0.5 pad 2.18)
  other vias: 42.9,22.63
N$73  (via drill 0.5 pad 2.18)
  other vias: 37.85,22.66
N$74  (via drill 0.5 pad 2.18)
  other vias: 35.33,22.66
N$75  (via drill 0.5 pad 2.18)
  other vias: 32.77,22.63
N$76  (via drill 0.5 pad 2.18)
  other vias: 30.25,22.63
N$77  (via drill 0.5 pad 2.18)
  other vias: 27.71,22.66
N$78  (via drill 0.5 pad 2.18)
  other vias: 25.17,22.66
N$79  (via drill 0.5 pad 2.18)
  other vias: 22.61,22.63
N$80  (via drill 0.5 pad 2.18)
  other vias: 65.81,37.87
N$81  (via drill 0.5 pad 2.18)
  other vias: 55.63,37.9
N$82  (via drill 0.5 pad 2.18)
  other vias: 53.09,37.9
N$83  (via drill 0.5 pad 2.18)
  other vias: 50.55,37.87
N$84  (via drill 0.5 pad 2.18)
  other vias: 48.01,37.9
N$85  (via drill 0.5 pad 2.18)
  other vias: 45.44,37.87
N$86  (via drill 0.5 pad 2.18)
  other vias: 42.9,37.85
N$87  (via drill 0.5 pad 2.18)
  other vias: 37.85,37.87
N$88  (via drill 0.5 pad 2.18)
  other vias: 35.28,37.85
N$89  (via drill 0.5 pad 2.18)
  other vias: 30.2,37.92
N$90  (via drill 0.5 pad 2.18)
  other vias: 27.69,37.87
N$91  (via drill 0.5 pad 2.18)
  other vias: 20.09,37.85
N$92  (via drill 0.5 pad 2.18)
  other vias: 17.55,37.87
N$93
  Bottom 0.61: 60.35,37.16 60.27,37.16 60.22,37.11 60.22,38.58 61.37,38.58
  Bottom 0.813: 60.76,38.43 61.27,38.43 61.27,37.16 60.35,37.16
N$94
  Bottom 0.61: 58.09,37.21 58.09,37.06 58.12,37.03 | 58.12,37.03 58.04,37.03 | 58.04,37.03 57.51,37.03 57.51,38.58 58.65,38.58 58.65,37.11 58.6,37.06 58.01,37.06 58.04,37.03 | 58.12,37.03 58.14,37.03 | 58.65,37.03 58.14,37.03 | 58.14,37.03 57.99,37.19 57.79,37.19 57.63,37.34 58.5,37.34 58.5,38.3 58.47,38.33 57.81,38.33 57.79,38.35 57.79,38.25 57.58,38.05 57.58,38.28 57.56,38.3
N$95
  Bottom 0.61: 57.71,38.48 57.71,37.44
N$96
  Bottom 0.61: 22.61,38.46 22.61,38.58 22.58,38.61 | 22.58,38.61 23.06,38.61 23.09,38.63 23.09,38.61 | 23.09,38.61 23.09,37.06 23.06,37.03 22.1,37.03 22.07,37.06 21.87,37.06 21.84,37.03 21.84,38.53 22.23,38.53 22.33,38.63 | 22.33,38.63 22.02,38.63 | 22.02,38.63 21.87,38.63 21.84,38.61 22.02,38.61 | 22.02,38.61 22.58,38.61 | 22.02,38.61 22.02,38.63 | 22.33,38.63 23.06,38.63 23.09,38.61
N$97
  Bottom 0.61: 24.82,38.18 25.43,38.18 25.48,38.23 25.48,38.28 25.43,38.33 25.53,38.33 25.71,38.15 25.71,37.39 25.63,37.31 24.97,37.31 24.82,37.16 25.1,37.16 25.15,37.11 25.25,37.11 25.27,37.08
N$98
  Bottom 0.61: 24.74,38.58 25.78,38.58 25.81,38.61 24.64,38.61 24.61,38.58 24.61,37.06 24.64,37.03 25.78,37.03 25.78,37.16 25.81,37.19 25.81,38.58 25.04,38.58 25.04,38.48
N$99
  Bottom 0.61: 22.94,37.36 22.2,37.36 22.15,37.31 22.15,38.12 22.1,38.18 22.1,37.57 21.97,37.44
N$100
  Bottom 1.016: 15.77,48.95 16.15,48.95 16.15,51.84 15.82,51.84 15.82,51.33 15.21,51.33 15.21,51.31 15.16,51.31 15.16,48.87 16.18,48.87 16.18,51.77
N$101
  Bottom 1.016: 23.32,50.19 23.34,50.19 23.34,51.23
N$102
  Bottom 1.016: 18.67,51.16 18.72,51.16 18.72,51.21 18.26,51.21 | 18.24,50.09 18.26,50.09 18.26,51.21 | 18.26,51.21 17.93,51.21 | 18.75,51.18 18.75,48.82 17.65,48.82 17.65,51.21 17.93,51.21 | 17.93,51.21 17.93,49.91 18.06,49.91 18.06,49.68
N$103
  Bottom 1.016: 20.75,50.09 21.26,50.09 21.26,49.1 21.29,49.1 21.29,50.98 | 20.83,50.98 21.29,50.98 | 21.29,50.98 21.29,51.21 20.27,51.21 20.27,48.84 21.31,48.84 21.31,49.17
N$104
  Bottom 1.016: 23.29,51.18 23.32,51.18 23.32,51.23 22.78,51.23 22.78,48.82 23.83,48.82 23.83,51.18 23.47,51.18 23.47,51.23 23.9,51.23 23.9,48.82 23.6,48.82 23.6,49.2
N$105
  Bottom 1.016: 25.86,49.86 25.83,49.86 25.83,51.18 26.39,51.18 26.39,48.84 26.37,48.84 26.37,48.79 25.32,48.79 25.32,51.66 26.44,51.66 26.44,51.74 26.42,51.74 | 26.42,51.74 26.42,51.08 26.42,48.87 26.19,48.87 26.19,50.04 | 26.42,51.74 26.42,52.12
N$106
  Bottom 1.016: 28.47,50.14 28.47,51.21 28.45,51.23 27.76,51.23 27.74,51.21 27.74,48.82 27.76,48.79 28.93,48.79 28.93,51.21 27.94,51.21 27.79,51.05 28.42,51.05 28.6,51.23 28.96,51.23 28.98,51.21 28.96,51.21 | 28.96,51.21 28.88,51.21 28.4,50.72 28.47,50.72 28.96,51.21 | 28.96,51.21 28.96,49.48 | 28.96,48.79 28.96,49.48 | 28.96,49.48 28.65,49.78
N$107
  Bottom 0.813: 41.2,49.99 41.2,51.21 41.1,51.31
N$108
  Bottom 0.813: 25.1,52.73 25.2,52.73 25.2,51.89 26.54,51.89 26.54,52.53 26.11,52.53 26.11,52.4
N$109
  Bottom 0.813: 43.18,51.11 43.16,51.11 43.16,51.33 | 44.3,51.23 44.3,51.33 43.16,51.33 | 44.3,51.23 44.27,51.23 44.27,48.77 44.3,48.77 44.3,48.69 43,48.69 43,51.31 42.98,51.31 42.98,51.33 43.16,51.33 | 44.3,51.23 44.3,48.79
N$110
  Bottom 0.813: 40.46,51.31 40.46,48.69 41.68,48.69 41.68,51.31 40.74,51.31 40.74,51.33 | 41.1,50.16 41.1,51.33 | 41.1,51.33 40.74,51.33 | 40.74,51.33 40.46,51.33 40.44,51.31 | 41.1,51.33 41.66,51.33 41.66,51.16 41.22,51.16 41.22,51.03
N$111
  Bottom 0.813: 46.2,50.11 45.64,50.11 45.64,51.28 45.62,51.28 45.62,51.31 45.64,51.31 | 45.75,51.31 45.64,51.31 | 45.64,51.31 45.64,51.33 46.66,51.33 46.66,49.15 45.64,49.15 | 45.64,49.15 45.64,50.01 | 45.64,49.15 45.64,48.74 46,48.74 46.66,49.12 46.23,49.61
N$112
  Bottom 0.406: 4.39,46.58 5,46.58 5,47.3 3.63,47.3 3.63,46.71 | 3.63,46.71 3.63,46.15 | 3.63,46.71 3.66,46.71 3.66,46.1 3.63,46.1 3.63,46.02 5.03,46.02 5.03,47.45 3.63,47.45 3.63,47.42 3.61,47.42 3.61,46.02 4.04,46.02 4.04,46.84
N$113
  Bottom 0.406: 18.67,46.66 18.59,46.66 18.59,46.1 20.02,46.1 20.02,47.35 18.59,47.35 18.59,47.04
N$114
  Bottom 0.406: 35.59,41.38 35.56,41.38 35.56,41.94 36.2,41.94 36.2,40.82 34.85,40.82 34.85,41.78 35.28,41.78 35.28,41.35
N$115
  Bottom 0.813: 16,51.87 16.28,51.87 16.28,52.81 16.08,52.81 16.08,52.58

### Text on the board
Bottom: elektronic.cekuj.net | LCDskop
